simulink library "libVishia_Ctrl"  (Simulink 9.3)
settings: Solver=ode45  StartTime=0.0  StopTime=10.0  RelTol=1e-3  EnableMultiTasking=on
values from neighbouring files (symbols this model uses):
  Tstep = 0.0001    [InspcCtrl_init.m]    (also in TestOrthOscObjO_init.m = 0.0005; stimuli_Smlk.m = 0.001; TestOrthOsc_init.m = 5e-05; Test_PIDctrl_init.m)
undefined symbols (not defined in the file or in its folder): Fmax, Fmin, Fnom, init, K, lim, maxError, minMagn, T1, Td, Tg, TP, Tstep_, y0
libraries: $bdroot x14, libVishia_Conv x8, simulink x5, lib_Inspc x1

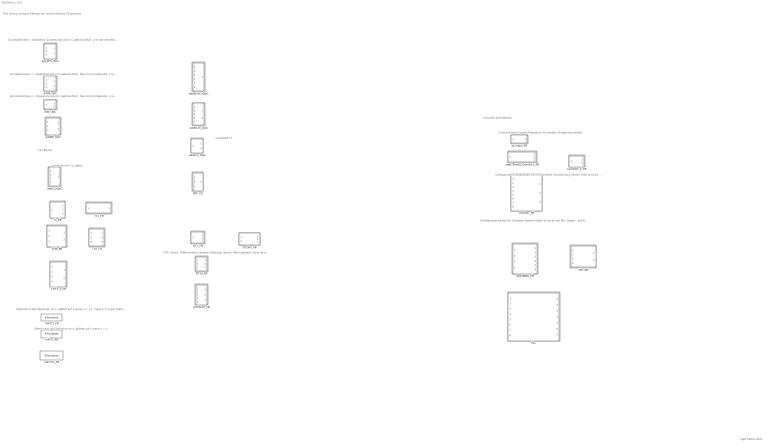
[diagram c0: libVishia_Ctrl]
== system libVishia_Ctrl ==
  note: right botton 60%
  note: Converts from a given Frequency to number of steps per period
  note: Simulink-pure Moduls
  note: This library contains FBlocks for control without S-Functions
  note: Orthogonaloszillator für 3-phasen-System Input ist als ab mit Mit- Gegen- und Nullsystem gegeben. Orthi separiert Gleichanteil (yG), Mitsystem(yM) und Gegensystem (yN) date=2016-03-04
  note: OrthogonalOscillator Basic-FB mit korrekter Rückführung. Dieser Orthi wird als Basis in den anderen FB verwendet.
  note: Grundglied des += Operators wie in C gebräuchlich. Das ist ein Integrator. y ist der neueste Wert. yz ist der gespeicherte Wert (Abarbeitung bevor +=). Ohne Setz-Möglichkeit. Initialwert als Parameter.
  note: Grundglied des += Operators wie in C gebräuchlich. Das ist ein Integrator. y ist der neueste Wert. yz ist der gespeicherte Wert (Abarbeitung bevor +=). Setzen: Wird in C häufig an anderer Stelle ausgeführt.
  note: Grundglied des = Operators (Zuweisung) wie in C gebräuchlich. y ist der neueste Wert, entweder =X oder =XS. yz ist der gespeicherte Wert. Setzen: Wird in C häufig an anderer Stelle ausgeführt.
  note: Variante mit z-1 außen.
  note: T1-FBlocks
  note: Übernimmt das Maximum an x, glättet auf x wenn x < y 1. Input x, 2. Input Faktor zum Glätten
  note: Übernimmt das Minimum an x, glättet auf x wenn x > y
  note: Limitated T1
  note: DT1 classic: Differenzierer, danach Glättung. Vorteil: Wenn gesetzt, dann ist das Differnzial 0
  DFF_CE : Subsystem
  DT1SLim_FB : Subsystem
  DT1S_FB : Subsystem
  DT1_FB : Subsystem
  DT1lim_FB : Subsystem
  OrthOsc_FB : Subsystem
  OrthiMNG_FB : Subsystem
  PLL : Subsystem
  T11_FB : Subsystem
  T1D_FB : Subsystem
  T1_FB : Subsystem
  T1fS_FB : Subsystem
  T1fT1_S_FB : Subsystem
  abn2pq : Subsystem
  addLim_OpC : Subsystem
  addSE_OpC : Subsystem  TreatAsAtomicUnit=on
  addSLim_OpC : Subsystem
  addSLim_zOpC : Subsystem
  addS_OpC : Subsystem
  addS_zOpC : Subsystem
  add_OpC : Subsystem
  assignS_OpC : Subsystem
  calcOrthi_fi_FB : Subsystem
  fq_steps_FB : Subsystem
  maxT1_FB : S-Function  FunctionName=maxT1_FB  Parameters=SampleTime  SFunctionDeploymentMode=off  EnableBusSupport=off
  maxnT1_FB : S-Function  FunctionName=maxnT1_FB  Parameters=SampleTime  SFunctionDeploymentMode=off  EnableBusSupport=off
  minT1_FB : S-Function  FunctionName=minT1_FB  Parameters=SampleTime  SFunctionDeploymentMode=off  EnableBusSupport=off
  step7Period_OrthOsc1_FB : Subsystem

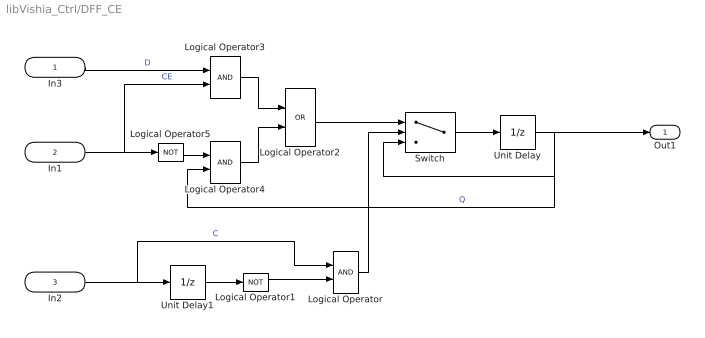
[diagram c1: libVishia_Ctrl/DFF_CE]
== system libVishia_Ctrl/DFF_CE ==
  In3 : Inport
  In1 : Inport  Port=2
  In2 : Inport  Port=3
  Logical Operator : Logic  IconShape=distinctive  AllPortsSameDT=off  OutDataTypeStr=boolean
  Logical Operator1 : Logic  Operator=NOT  IconShape=distinctive  AllPortsSameDT=off  OutDataTypeStr=boolean
  Logical Operator2 : Logic  Operator=OR  IconShape=distinctive  AllPortsSameDT=off  OutDataTypeStr=boolean
  Logical Operator3 : Logic  IconShape=distinctive  AllPortsSameDT=off  OutDataTypeStr=boolean
  Logical Operator4 : Logic  IconShape=distinctive  AllPortsSameDT=off  OutDataTypeStr=boolean
  Logical Operator5 : Logic  Operator=NOT  IconShape=distinctive  AllPortsSameDT=off  OutDataTypeStr=boolean
  Switch : Switch  Criteria=u2 > Threshold
  Unit Delay : UnitDelay  SampleTime=-1  HasFrameUpgradeWarning=on
  Unit Delay1 : UnitDelay  SampleTime=-1  HasFrameUpgradeWarning=on
  Out1 : Outport  OutDataTypeStr=boolean
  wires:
  In1/1 -> Logical Operator3/2, Logical Operator5/1  "CE"
  Switch/1 -> Unit Delay/1
  In2/1 -> Logical Operator/1, Unit Delay1/1  "C"
  Unit Delay1/1 -> Logical Operator1/1
  Logical Operator1/1 -> Logical Operator/2
  Logical Operator/1 -> Switch/2
  Unit Delay/1 -> Logical Operator4/2, Switch/3, Out1/1  "Q"
  In3/1 -> Logical Operator3/1  "D"
  Logical Operator5/1 -> Logical Operator4/1
  Logical Operator2/1 -> Switch/1
  Logical Operator4/1 -> Logical Operator2/2
  Logical Operator3/1 -> Logical Operator2/1

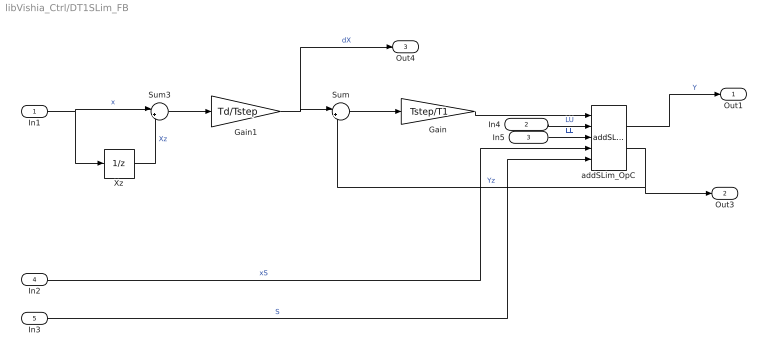
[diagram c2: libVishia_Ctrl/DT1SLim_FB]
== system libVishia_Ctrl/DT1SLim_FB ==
  In1 : Inport
  In4 : Inport  Port=2
  In5 : Inport  Port=3
  In2 : Inport  Port=4
  In3 : Inport  Port=5
  Gain : Gain  Gain=Tstep/T1
  Gain1 : Gain  Gain=Td/Tstep
  Sum : Sum  Inputs=|+-
  Sum3 : Sum  Inputs=|+-
  Xz : UnitDelay  SampleTime=Tstep  HasFrameUpgradeWarning=on
  addSLim_OpC : $bdroot/addSLim_OpC  y0=0  Tstep=Tstep
  Out1 : Outport
  Out3 : Outport  Port=2
  Out4 : Outport  Port=3
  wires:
  addSLim_OpC/2 -> Out3/1, Sum/2  "Yz"
  In3/1 -> addSLim_OpC/5  "S"
  In2/1 -> addSLim_OpC/4  "xS"
  Sum3/1 -> Gain1/1
  Xz/1 -> Sum3/2  "Xz"
  Gain1/1 -> Sum/1, Out4/1  "dX"
  addSLim_OpC/1 -> Out1/1  "Y"
  In1/1 -> Sum3/1, Xz/1  "x"
  Sum/1 -> Gain/1
  Gain/1 -> addSLim_OpC/1
  In4/1 -> addSLim_OpC/2  "LU"
  In5/1 -> addSLim_OpC/3  "LL"

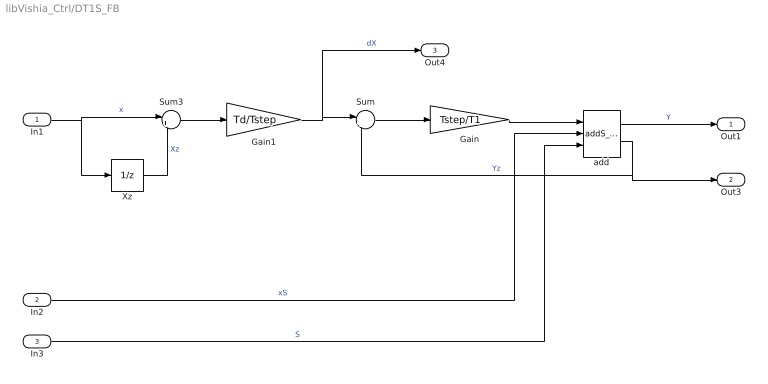
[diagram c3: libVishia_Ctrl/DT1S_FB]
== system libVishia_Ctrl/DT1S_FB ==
  In1 : Inport
  In2 : Inport  Port=2
  In3 : Inport  Port=3
  Gain : Gain  Gain=Tstep/T1
  Gain1 : Gain  Gain=Td/Tstep
  Sum : Sum  Inputs=|+-
  Sum3 : Sum  Inputs=|+-
  Xz : UnitDelay  SampleTime=Tstep  HasFrameUpgradeWarning=on
  add : $bdroot/addS_OpC  init=0  Tstep=Tstep
  Out1 : Outport
  Out3 : Outport  Port=2
  Out4 : Outport  Port=3
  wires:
  Gain/1 -> add/1
  Sum/1 -> Gain/1
  In1/1 -> Xz/1, Sum3/1  "x"
  add/1 -> Out1/1  "Y"
  Gain1/1 -> Out4/1, Sum/1  "dX"
  Xz/1 -> Sum3/2  "Xz"
  Sum3/1 -> Gain1/1
  In2/1 -> add/2  "xS"
  In3/1 -> add/3  "S"
  add/2 -> Sum/2, Out3/1  "Yz"

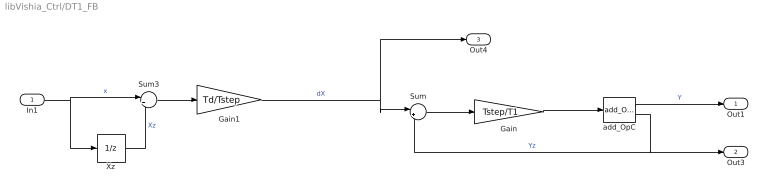
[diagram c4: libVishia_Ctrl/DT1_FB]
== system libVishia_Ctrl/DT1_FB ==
  In1 : Inport
  Gain : Gain  Gain=Tstep/T1
  Gain1 : Gain  Gain=Td/Tstep
  Sum : Sum  Inputs=|+-
  Sum3 : Sum  Inputs=|+-
  Xz : UnitDelay  SampleTime=Tstep  HasFrameUpgradeWarning=on
  add_OpC : $bdroot/add_OpC  y0=0  Tstep=Tstep
  Out1 : Outport
  Out3 : Outport  Port=2
  Out4 : Outport  Port=3
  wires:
  add_OpC/2 -> Out3/1, Sum/2  "Yz"
  Sum3/1 -> Gain1/1
  Xz/1 -> Sum3/2  "Xz"
  add_OpC/1 -> Out1/1  "Y"
  In1/1 -> Sum3/1, Xz/1  "x"
  Sum/1 -> Gain/1
  Gain/1 -> add_OpC/1
  Gain1/1 -> Sum/1, Out4/1  "dX"

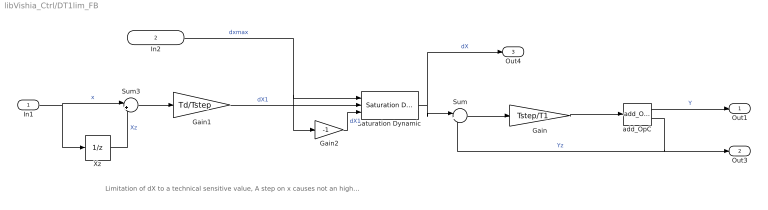
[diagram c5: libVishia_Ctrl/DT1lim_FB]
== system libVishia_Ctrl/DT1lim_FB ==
  note: Limitation of dX to a technical sensitive value, A step on x causes not an higher value on dX1, which is smoothed. So fast changes are filtered.
  In1 : Inport
  In2 : Inport  Port=2
  Gain : Gain  Gain=Tstep/T1
  Gain1 : Gain  Gain=Td/Tstep
  Gain2 : Gain  Gain=-1
  Saturation Dynamic : simulink/Discontinuities/Saturation Dynamic  OutMin=[]  OutMax=[]  OutDataTypeStr=Inherit: Same as second input  OutDataType=fixdt(1, 16)  OutScaling=2^-10  DoSatur=off
  Sum : Sum  Inputs=|+-
  Sum3 : Sum  Inputs=|+-
  Xz : UnitDelay  SampleTime=Tstep  HasFrameUpgradeWarning=on
  add_OpC : $bdroot/add_OpC  y0=0  Tstep=Tstep
  Out1 : Outport
  Out3 : Outport  Port=2
  Out4 : Outport  Port=3
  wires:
  Saturation Dynamic/1 -> Out4/1, Sum/1  "dX"
  Gain/1 -> add_OpC/1
  Sum/1 -> Gain/1
  In1/1 -> Xz/1, Sum3/1  "x"
  add_OpC/1 -> Out1/1  "Y"
  Gain1/1 -> Saturation Dynamic/2  "dX1"
  Xz/1 -> Sum3/2  "Xz"
  Sum3/1 -> Gain1/1
  add_OpC/2 -> Sum/2, Out3/1  "Yz"
  In2/1 -> Gain2/1, Saturation Dynamic/1  "dxmax"
  Gain2/1 -> Saturation Dynamic/3  "dX1"

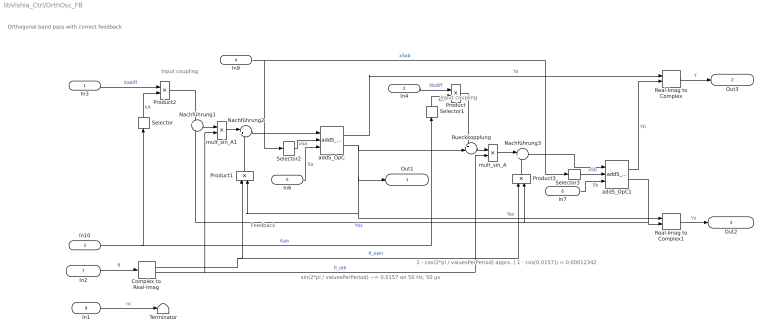
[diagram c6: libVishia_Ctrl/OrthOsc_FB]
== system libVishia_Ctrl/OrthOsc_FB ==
  note: 1 - cos(2*pi / valuesPerPeriod) apprx. ( 1 - cos(0.0157)) = 0.00012342
  note: Input coupling
  note: Feedback
  note: sin(2*pi / valuesPerPeriod) ~= 0.0157 on 50 Hz, 50 µs
  note: Orthogonal band pass with correct feedback
  note: Input coupling
  In3 : Inport
  In4 : Inport  Port=2
  In10 : Inport  Port=3  OutDataTypeStr=single  PortDimensions=2
  In9 : Inport  Port=4
  In6 : Inport  Port=5  OutDataTypeStr=boolean
  In7 : Inport  Port=6  OutDataTypeStr=boolean
  In2 : Inport  Port=7  OutDataTypeStr=single
  In1 : Inport  Port=8  OutDataTypeStr=boolean
  Complex to Real-Imag : ComplexToRealImag
  Nachführung1 : Sum  Inputs=+|-
  Nachführung2 : Sum  Inputs=|+-
  Nachführung3 : Sum  Inputs=|+-
  Product{,1..3} (4 alike) : Product
  Real-Imag to Complex : RealImagToComplex
  Real-Imag to Complex1 : RealImagToComplex
  Rueckkopplung : Sum  Inputs=++|
  Selector : Selector  InputPortWidth=2  IndexOptions=Index vector (dialog)  Indices=[1]  OutputSizes=1
  Selector1 : Selector  InputPortWidth=2  IndexOptions=Index vector (dialog)  Indices=[2]  OutputSizes=1
  Selector2 : Selector  InputPortWidth=2  IndexOptions=Index vector (dialog)  Indices=[1]  OutputSizes=1
  Selector3 : Selector  InputPortWidth=2  IndexOptions=Index vector (dialog)  Indices=[2]  OutputSizes=1
  Terminator : Terminator
  addS_OpC : $bdroot/addS_OpC  init=0  Tstep=-1
  addS_OpC1 : $bdroot/addS_OpC  init=0  Tstep=-1
  mult_sin_A : Product
  mult_sin_A1 : Product
  Out1 : Outport
  Out3 : Outport  Port=2
  Out2 : Outport  Port=3
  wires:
  Complex to Real-Imag/2 -> mult_sin_A1/2, mult_sin_A/2  "fI_oth"
  Real-Imag to Complex/1 -> Out3/1  "Y"
  mult_sin_A1/1 -> Nachführung2/1
  Nachführung1/1 -> mult_sin_A1/1
  addS_OpC/2 -> Out1/1, Real-Imag to Complex1/1, Product1/2, Rueckkopplung/2  "Yaz"
  Product2/1 -> Nachführung1/1
  In3/1 -> Product2/1  "Xadiff"
  Product/1 -> Rueckkopplung/1
  In2/1 -> Complex to Real-Imag/1  "fI"
  Rueckkopplung/1 -> mult_sin_A/1
  mult_sin_A/1 -> Nachführung3/1
  addS_OpC/1 -> Real-Imag to Complex/1  "Ya"
  addS_OpC1/2 -> Nachführung1/2, Product3/2, Real-Imag to Complex1/2  "Ybz"
  Selector/1 -> Product2/2  "kA"
  In6/1 -> addS_OpC/3  "Sa"
  In4/1 -> Product/1  "Xbdiff"
  Selector1/1 -> Product/2  "kB"
  In7/1 -> addS_OpC1/3  "Sb"
  Selector3/1 -> addS_OpC1/2  "xSb"
  Selector2/1 -> addS_OpC/2  "xSA"
  Nachführung2/1 -> addS_OpC/1
  Product1/1 -> Nachführung2/2
  Nachführung3/1 -> addS_OpC1/1
  Product3/1 -> Nachführung3/2
  Complex to Real-Imag/1 -> Product1/1, Product3/1  "fI_own"
  addS_OpC1/1 -> Real-Imag to Complex/2  "Yb"
  Real-Imag to Complex1/1 -> Out2/1  "Yz"
  In10/1 -> Selector/1, Selector1/1  "Kab"
  In9/1 -> Selector3/1, Selector2/1  "xSab"
  In1/1 -> Terminator/1  "nc"

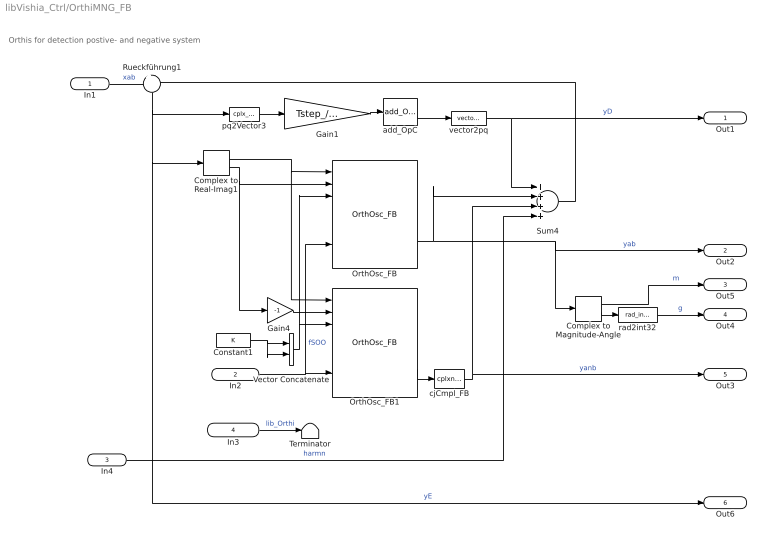
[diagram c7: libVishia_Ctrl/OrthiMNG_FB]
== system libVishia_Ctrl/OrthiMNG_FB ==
  note: Orthis for detection postive- and negative system
  In1 : Inport  OutDataTypeStr=single
  In2 : Inport  Port=2  OutDataTypeStr=single
  In4 : Inport  Port=3  OutDataTypeStr=single
  In3 : Inport  Port=4  OutDataTypeStr=boolean
  Complex to Magnitude-Angle : ComplexToMagnitudeAngle
  Complex to Real-Imag1 : ComplexToRealImag
  Constant1 : Constant  Value=K  OutDataTypeStr=single
  Gain1 : Gain  Gain=Tstep_/Tg
  Gain4 : Gain  Gain=-1
  OrthOsc_FB : $bdroot/OrthOsc_FB
  OrthOsc_FB1 : $bdroot/OrthOsc_FB
  Rueckführung1 : Sum  Inputs=+-
  Sum4 : Sum  Inputs=++++
  Terminator : Terminator
  Vector Concatenate : Concatenate
  add_OpC : $bdroot/add_OpC  y0=0  Tstep=-1
  cjCmpl_FB : libVishia_Conv/cplxni_FB  SystemSampleTime=-1
  pq2Vector3 : libVishia_Conv/cplx_vector_FB  SystemSampleTime=-1
  rad2int32 : libVishia_Conv/rad_int32_FB  SystemSampleTime=-1
  vector2pq : libVishia_Conv/vector_cplx_FB  SystemSampleTime=-1
  Out1 : Outport  OutDataTypeStr=single
  Out2 : Outport  Port=2  OutDataTypeStr=single
  Out5 : Outport  Port=3  OutDataTypeStr=single
  Out4 : Outport  Port=4  OutDataTypeStr=int32
  Out3 : Outport  Port=5  OutDataTypeStr=single
  Out6 : Outport  Port=6  OutDataTypeStr=single
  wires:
  In4/1 -> Sum4/4  "harmn"
  In3/1 -> Terminator/1  "lib_Orthi"
  Constant1/1 -> Vector Concatenate/1, Vector Concatenate/2
  Gain4/1 -> OrthOsc_FB1/2
  Complex to Real-Imag1/2 -> OrthOsc_FB/2, Gain4/1
  add_OpC/2 -> vector2pq/1
  pq2Vector3/1 -> Gain1/1
  Complex to Real-Imag1/1 -> OrthOsc_FB/1, OrthOsc_FB1/1
  vector2pq/1 -> Out1/1, Sum4/1  "yD"
  Vector Concatenate/1 -> OrthOsc_FB/3, OrthOsc_FB1/3
  Rueckführung1/1 -> pq2Vector3/1, Complex to Real-Imag1/1, Out6/1  "yE"
  In1/1 -> Rueckführung1/1  "xab"
  Gain1/1 -> add_OpC/1
  In2/1 -> OrthOsc_FB1/7, OrthOsc_FB/7  "fSOO"
  OrthOsc_FB/3 -> Complex to Magnitude-Angle/1, Out2/1, Sum4/2  "yab"
  Sum4/1 -> Rueckführung1/2
  cjCmpl_FB/1 -> Out3/1, Sum4/3  "yanb"
  OrthOsc_FB1/3 -> cjCmpl_FB/1
  Complex to Magnitude-Angle/2 -> rad2int32/1
  rad2int32/1 -> Out4/1  "g"
  Complex to Magnitude-Angle/1 -> Out5/1  "m"

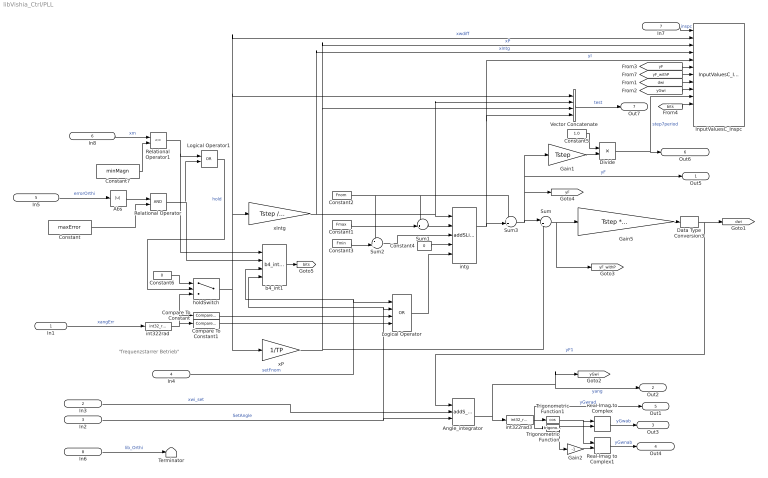
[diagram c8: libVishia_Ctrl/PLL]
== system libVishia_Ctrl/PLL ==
  note: "frequenzstarrer Betrieb"
  In1 : Inport
  In3 : Inport  Port=2  OutDataTypeStr=int32
  In2 : Inport  Port=3  OutDataTypeStr=boolean
  In4 : Inport  Port=4  OutDataTypeStr=boolean
  In5 : Inport  Port=5  OutDataTypeStr=single  PortDimensions=1
  In8 : Inport  Port=6  OutDataTypeStr=single  PortDimensions=1
  In7 : Inport  Port=7  OutDataTypeStr=uint32  PortDimensions=1  SampleTime=Tstep
  In6 : Inport  Port=8  OutDataTypeStr=boolean
  Abs : Abs
  Angle_integrator : $bdroot/addS_OpC  init=0  Tstep=-1
  Compare To Constant : simulink/Logic and Bit Operations/Compare To Constant  relop=>=  const=0.1  OutDataTypeStr=boolean
  Compare To Constant1 : simulink/Logic and Bit Operations/Compare To Constant  relop=<  const=-0.1  OutDataTypeStr=boolean
  Constant : Constant  Value=maxError
  Constant1 : Constant  Value=Fmax  OutDataTypeStr=single
  Constant2 : Constant  Value=Fnom  OutDataTypeStr=single
  Constant3 : Constant  Value=Fmin  OutDataTypeStr=single
  Constant4 : Constant  Value=0  OutDataTypeStr=single
  Constant5 : Constant  Value=1.0  OutDataTypeStr=single
  Constant6 : Constant  Value=0  OutDataTypeStr=single
  Constant7 : Constant  Value=minMagn
  Data Type Conversion3 : DataTypeConversion  OutDataTypeStr=int32
  Divide : Product  Inputs=*/
  Gain1 : Gain  Gain=Tstep
  Gain2 : Gain  Gain=-1
  Gain5 : Gain  Gain=Tstep * 65536 * 65536
  InputValuesC_Inspc : lib_Inspc/InputValuesC_Inspc  Commented=on  nameRefl=nameInspc  n1='wxdiff_rad'  n2='xP'  n3='xIntg'  n4='yIntg'  n5='yF'  n6='yF_withP'  n7='dwi'  n8='yGwi'  n9='step7period'  n10='hold_setG_setF_err_magn'  n11=''  n12=''
  Logical Operator : Logic  Operator=OR  Inputs=4  IconShape=distinctive  AllPortsSameDT=off  OutDataTypeStr=boolean
  Logical Operator1 : Logic  Operator=OR  AllPortsSameDT=off  OutDataTypeStr=boolean
  Real-Imag to Complex : RealImagToComplex
  Real-Imag to Complex1 : RealImagToComplex
  Relational Operator : RelationalOperator  OutDataTypeStr=boolean
  Relational Operator1 : RelationalOperator  Operator=<=  OutDataTypeStr=boolean
  Sum : Sum  Inputs=|++
  Sum1 : Sum  Inputs=-+|
  Sum2 : Sum  Inputs=-+|
  Sum3 : Sum  Inputs=++|
  Terminator : Terminator
  Trigonometric Function : Trigonometry
  Trigonometric Function1 : Trigonometry  Operator=cos
  Vector Concatenate : Concatenate  NumInputs=4
  b4_int1 : libVishia_Conv/b4_int32_FB  b0bit=0  b1bit=1  b2bit=2  b3bit=3
  holdSwitch : Switch
  int322rad : libVishia_Conv/int32_rad_FB  SystemSampleTime=-1
  int322rad3 : libVishia_Conv/int32_rad_FB  SystemSampleTime=-1
  intg : $bdroot/addSLim_OpC  y0=0  Tstep=-1
  xIntg : Gain  Gain=Tstep / Tintg
  xP : Gain  Gain=1/TP
  Out5 : Outport  OutDataTypeStr=single  PortDimensions=1
  Out2 : Outport  Port=2  OutDataTypeStr=int32  PortDimensions=1
  Out3 : Outport  Port=3  OutDataTypeStr=single  PortDimensions=1
  Out4 : Outport  Port=4  OutDataTypeStr=single  PortDimensions=1
  Out1 : Outport  Port=5  OutDataTypeStr=single  PortDimensions=1
  Out6 : Outport  Port=6  OutDataTypeStr=single  PortDimensions=1
  Out7 : Outport  Port=7  OutDataTypeStr=single  PortDimensions=4
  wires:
  [bits] -> InputValuesC_Inspc/11
  b4_int1/1 -> [bits]
  [yF] -> InputValuesC_Inspc/6
  In8/1 -> Relational Operator1/1  "xm"
  Relational Operator/1 -> b4_int1/2, Logical Operator1/2
  Relational Operator1/1 -> b4_int1/1, Logical Operator1/1
  Constant7/1 -> Relational Operator1/2
  Constant/1 -> Relational Operator/2
  Abs/1 -> Relational Operator/1
  In5/1 -> Abs/1  "errorOrthi"
  [yGwi] -> InputValuesC_Inspc/9
  [dwi] -> InputValuesC_Inspc/8
  [yF_withP] -> InputValuesC_Inspc/7
  In7/1 -> InputValuesC_Inspc/1  "inspc"
  int322rad/1 -> Compare To Constant1/1, holdSwitch/3, Compare To Constant/1
  Constant6/1 -> holdSwitch/1
  Vector Concatenate/1 -> Out7/1  "test"
  In6/1 -> Terminator/1  "lib_Orthi"
  holdSwitch/1 -> Vector Concatenate/1, InputValuesC_Inspc/2, xIntg/1, xP/1  "xwdiff"
  Logical Operator1/1 -> holdSwitch/2  "hold"
  In4/1 -> Logical Operator/1, b4_int1/3  "setFnom"
  Logical Operator/1 -> intg/5
  Divide/1 -> Out6/1, InputValuesC_Inspc/10  "step7period"
  Constant5/1 -> Divide/1
  Gain1/1 -> Divide/2
  In3/1 -> Angle_integrator/2  "xwi_set"
  In2/1 -> b4_int1/4, Logical Operator/2, Angle_integrator/3  "SetAngle"
  xIntg/1 -> Vector Concatenate/2, intg/1, InputValuesC_Inspc/4  "xIntg"
  xP/1 -> Sum/2, Vector Concatenate/3, InputValuesC_Inspc/3  "xP"
  In1/1 -> int322rad/1  "xangErr"
  Constant4/1 -> intg/4
  Constant3/1 -> Sum2/2
  Sum2/1 -> intg/3
  Sum1/1 -> intg/2
  Constant2/1 -> Sum3/1, Sum1/1, Sum2/1
  Sum/1 -> Gain5/1, [yF_withP]
  Data Type Conversion3/1 -> Angle_integrator/1, [dwi]  "yF1"
  Constant1/1 -> Sum1/2
  intg/1 -> Sum3/2, Vector Concatenate/4, InputValuesC_Inspc/5  "yI"
  Gain5/1 -> Data Type Conversion3/1
  Real-Imag to Complex1/1 -> Out4/1  "yGwnab"
  Real-Imag to Complex/1 -> Out3/1  "yGwab"
  Gain2/1 -> Real-Imag to Complex1/2
  Trigonometric Function/1 -> Real-Imag to Complex/2, Gain2/1
  Trigonometric Function1/1 -> Real-Imag to Complex/1, Real-Imag to Complex1/1
  int322rad3/1 -> Trigonometric Function1/1, Trigonometric Function/1, Out1/1  "yGwrad"
  Angle_integrator/2 -> int322rad3/1, Out2/1, [yGwi]  "yang"
  Sum3/1 -> Out5/1, Gain1/1, [yF], Sum/1  "yF"
  Compare To Constant/1 -> Logical Operator/3
  Compare To Constant1/1 -> Logical Operator/4

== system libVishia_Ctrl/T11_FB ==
  note: Yz += Tstep/T1 * (x - Yz)
  In1 : Inport
  Gain : Gain  Gain=Tstep/T1
  Sum : Sum  Inputs=|+-
  Sum6 : Sum  Inputs=|++
  Unit Delay : UnitDelay  InitialCondition=y0  SampleTime=Tstep  HasFrameUpgradeWarning=on
  Out2 : Outport
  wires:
  In1/1 -> Sum/1  "X"
  Sum/1 -> Gain/1  "dT1_Y"
  Gain/1 -> Sum6/1
  Sum6/1 -> Unit Delay/1
  Unit Delay/1 -> Sum/2, Sum6/2, Out2/1  "y"

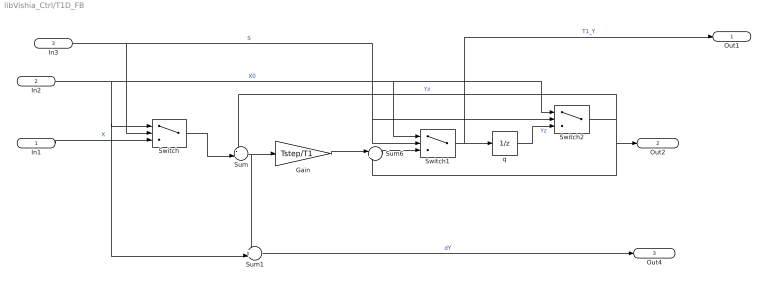
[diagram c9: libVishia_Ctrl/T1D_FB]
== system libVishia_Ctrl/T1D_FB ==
  In1 : Inport
  In2 : Inport  Port=2
  In3 : Inport  Port=3
  Gain : Gain  Gain=Tstep/T1
  Sum : Sum  Inputs=-+|
  Sum1 : Sum  Inputs=++|
  Sum6 : Sum  Inputs=|++
  Switch : Switch  Criteria=u2 ~= 0
  Switch1 : Switch  Criteria=u2 ~= 0
  Switch2 : Switch  Criteria=u2 ~= 0
  q : UnitDelay  InitialCondition=y0  SampleTime=Tstep  HasFrameUpgradeWarning=on
  Out1 : Outport
  Out2 : Outport  Port=2
  Out4 : Outport  Port=3
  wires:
  Switch2/1 -> Sum6/2, Out2/1, Sum/1  "Yz"
  Switch1/1 -> Out1/1, q/1  "T1_Y"
  In1/1 -> Switch/3  "X"
  In2/1 -> Sum1/2, Switch/1, Switch1/1, Switch2/1  "X0"
  Sum/1 -> Gain/1, Sum1/1
  In3/1 -> Switch/2, Switch2/2, Switch1/2  "S"
  Switch/1 -> Sum/2
  Sum1/1 -> Out4/1  "dY"
  Gain/1 -> Sum6/1
  Sum6/1 -> Switch1/3
  q/1 -> Switch2/3  "Yz"

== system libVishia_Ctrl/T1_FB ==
  note: Yz += Tstep/T1 * (x - Yz)
  In1 : Inport
  Gain : Gain  Gain=Tstep/T1
  Sum : Sum  Inputs=|+-
  add_OpC : $bdroot/add_OpC  y0=y0  Tstep=-1
  Out1 : Outport
  Out2 : Outport  Port=2
  Out4 : Outport  Port=3
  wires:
  Gain/1 -> add_OpC/1
  Sum/1 -> Out4/1, Gain/1  "dT1_Y"
  In1/1 -> Sum/1  "X"
  add_OpC/1 -> Out1/1  "T1_Y"
  add_OpC/2 -> Out2/1, Sum/2  "Yz"

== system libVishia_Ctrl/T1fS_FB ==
  In1 : Inport
  In2 : Inport  Port=2
  In3 : Inport  Port=3  OutDataTypeStr=boolean
  Gain : Gain  Gain=Tstep/T1
  Sum : Sum  Inputs=|+-
  addS_OpC : $bdroot/addS_OpC  init=init  Tstep=Tstep
  Out1 : Outport
  Out2 : Outport  Port=2
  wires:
  Gain/1 -> addS_OpC/1
  Sum/1 -> Gain/1
  In1/1 -> Sum/1  "x"
  addS_OpC/1 -> Out1/1  "Y"
  addS_OpC/2 -> Out2/1, Sum/2  "Yz"
  In2/1 -> addS_OpC/2  "xS"
  In3/1 -> addS_OpC/3  "S"

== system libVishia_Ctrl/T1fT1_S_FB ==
  In1 : Inport
  In4 : Inport  Port=2
  In2 : Inport  Port=3
  In3 : Inport  Port=4  OutDataTypeStr=boolean
  Gain : Gain  Gain=Tstep/T1
  Product : Product
  Sum : Sum  Inputs=|+-
  addS_OpC : $bdroot/addS_OpC  init=y0  Tstep=Tstep
  Out1 : Outport
  Out2 : Outport  Port=2
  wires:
  In3/1 -> addS_OpC/3  "S"
  In2/1 -> addS_OpC/2  "xS"
  addS_OpC/2 -> Sum/2, Out2/1  "Yz"
  addS_OpC/1 -> Out1/1  "Y_T1"
  In1/1 -> Sum/1  "x"
  Sum/1 -> Gain/1
  Product/1 -> addS_OpC/1
  In4/1 -> Product/1  "fT1"
  Gain/1 -> Product/2

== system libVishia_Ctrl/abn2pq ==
  note: Park transformation of positive and negativ system
  In1 : Inport  OutDataTypeStr=single
  In2 : Inport  Port=2  OutDataTypeStr=single
  In4 : Inport  Port=3  OutDataTypeStr=single
  In3 : Inport  Port=4  OutDataTypeStr=boolean
  Product : Product
  Product1 : Product
  Terminator : Terminator
  cplxni_FB : libVishia_Conv/cplxni_FB  SystemSampleTime=-1
  Out4 : Outport  OutDataTypeStr=single
  Out5 : Outport  Port=2  OutDataTypeStr=single
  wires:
  In3/1 -> Terminator/1  "lib_OrthOsc"
  In1/1 -> Product/1  "ab"
  In2/1 -> Product1/1  "abN"
  cplxni_FB/1 -> Product/2
  In4/1 -> cplxni_FB/1, Product1/2  "xgab"
  Product/1 -> Out4/1  "ypq"
  Product1/1 -> Out5/1  "ypqN"

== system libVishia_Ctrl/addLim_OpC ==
  x : Inport
  Saturation : Saturate  UpperLimit=lim  LowerLimit=-lim
  Sum6 : Sum  Inputs=|++
  Unit Delay : UnitDelay  InitialCondition=y0  SampleTime=Tstep  HasFrameUpgradeWarning=on
  y : Outport
  yz : Outport  Port=2
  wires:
  Unit Delay/1 -> Sum6/2, yz/1
  x/1 -> Sum6/1
  Saturation/1 -> y/1, Unit Delay/1
  Sum6/1 -> Saturation/1

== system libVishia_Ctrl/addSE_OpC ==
  x : Inport
  xS : Inport  Port=2
  S : Inport  Port=3  OutDataTypeStr=boolean
  Enable : EnablePort
  Sum6 : Sum  Inputs=|++
  Switch : Switch  Criteria=u2 ~= 0
  q : UnitDelay  SampleTime=-1  HasFrameUpgradeWarning=on
  y : Outport
  yz : Outport  Port=2
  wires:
  Switch/1 -> q/1, y/1
  x/1 -> Sum6/1
  q/1 -> Sum6/2, yz/1
  S/1 -> Switch/2
  Sum6/1 -> Switch/3
  xS/1 -> Switch/1

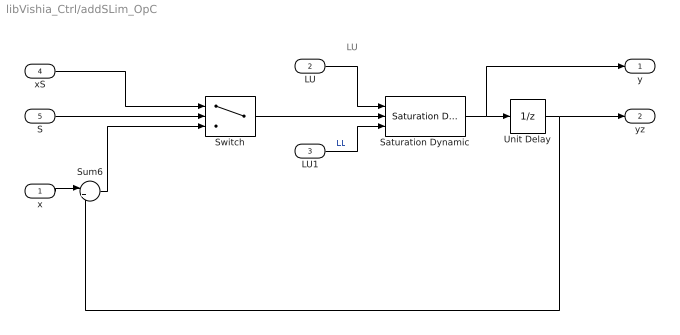
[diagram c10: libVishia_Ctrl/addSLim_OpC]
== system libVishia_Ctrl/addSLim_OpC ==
  note: LU
  x : Inport
  LU : Inport  Port=2
  LU1 : Inport  Port=3
  xS : Inport  Port=4
  S : Inport  Port=5  OutDataTypeStr=boolean
  Saturation Dynamic : simulink/Discontinuities/Saturation Dynamic  OutMin=[]  OutMax=[]  OutDataTypeStr=Inherit: Same as second input  OutDataType=fixdt(1, 16)  OutScaling=2^-10  DoSatur=off
  Sum6 : Sum  Inputs=|++
  Switch : Switch  Criteria=u2 ~= 0
  Unit Delay : UnitDelay  InitialCondition=y0  SampleTime=Tstep  HasFrameUpgradeWarning=on
  y : Outport
  yz : Outport  Port=2
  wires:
  Switch/1 -> Saturation Dynamic/2
  S/1 -> Switch/2
  Unit Delay/1 -> yz/1, Sum6/2
  xS/1 -> Switch/1
  x/1 -> Sum6/1
  Sum6/1 -> Switch/3
  Saturation Dynamic/1 -> y/1, Unit Delay/1
  LU/1 -> Saturation Dynamic/1
  LU1/1 -> Saturation Dynamic/3  "LL"

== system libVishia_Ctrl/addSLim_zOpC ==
  note: LU
  x : Inport
  LU : Inport  Port=2
  LU1 : Inport  Port=3
  xS : Inport  Port=4
  S : Inport  Port=5  OutDataTypeStr=boolean
  yz : Inport  Port=6
  Saturation Dynamic : simulink/Discontinuities/Saturation Dynamic  OutMin=[]  OutMax=[]  OutDataTypeStr=Inherit: Same as second input  OutDataType=fixdt(1, 16)  OutScaling=2^-10  DoSatur=off
  Sum6 : Sum  Inputs=|++
  Switch : Switch  Criteria=u2 ~= 0
  y : Outport
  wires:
  LU1/1 -> Saturation Dynamic/3  "LL"
  LU/1 -> Saturation Dynamic/1
  Saturation Dynamic/1 -> y/1  "y"
  Sum6/1 -> Switch/3
  x/1 -> Sum6/1
  xS/1 -> Switch/1
  S/1 -> Switch/2
  Switch/1 -> Saturation Dynamic/2
  yz/1 -> Sum6/2  "yz"

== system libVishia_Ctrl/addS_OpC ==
  x : Inport
  xS : Inport  Port=2
  S : Inport  Port=3  OutDataTypeStr=boolean
  Sum6 : Sum  Inputs=|++
  Switch : Switch  Criteria=u2 ~= 0
  q : UnitDelay  InitialCondition=init  SampleTime=Tstep  HasFrameUpgradeWarning=on
  y : Outport
  yz : Outport  Port=2
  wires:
  Sum6/1 -> Switch/3
  x/1 -> Sum6/1
  xS/1 -> Switch/1
  q/1 -> Sum6/2, yz/1
  S/1 -> Switch/2
  Switch/1 -> q/1, y/1

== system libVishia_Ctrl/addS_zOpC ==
  x : Inport
  xS : Inport  Port=2
  S : Inport  Port=3  OutDataTypeStr=boolean
  yz : Inport  Port=4
  Sum6 : Sum  Inputs=|++
  Switch : Switch  Criteria=u2 ~= 0
  y : Outport
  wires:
  Switch/1 -> y/1
  S/1 -> Switch/2
  xS/1 -> Switch/1
  x/1 -> Sum6/1
  Sum6/1 -> Switch/3
  yz/1 -> Sum6/2  "yz"

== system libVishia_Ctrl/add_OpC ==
  x : Inport
  Delay : Delay  DelayLength=1  InitialCondition=y0  SampleTime=Tstep
  Sum6 : Sum  Inputs=|++
  y : Outport
  yz : Outport  Port=2
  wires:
  Sum6/1 -> Delay/1, y/1
  x/1 -> Sum6/1
  Delay/1 -> Sum6/2, yz/1

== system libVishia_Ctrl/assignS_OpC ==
  x : Inport
  xS : Inport  Port=2
  S : Inport  Port=3  OutDataTypeStr=boolean
  Switch : Switch  Criteria=u2 ~= 0
  Unit Delay : UnitDelay  InitialCondition=y0  SampleTime=Tstep  HasFrameUpgradeWarning=on
  y : Outport
  yz : Outport  Port=2
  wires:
  Switch/1 -> y/1, Unit Delay/1
  S/1 -> Switch/2
  Unit Delay/1 -> yz/1
  xS/1 -> Switch/1
  x/1 -> Switch/3

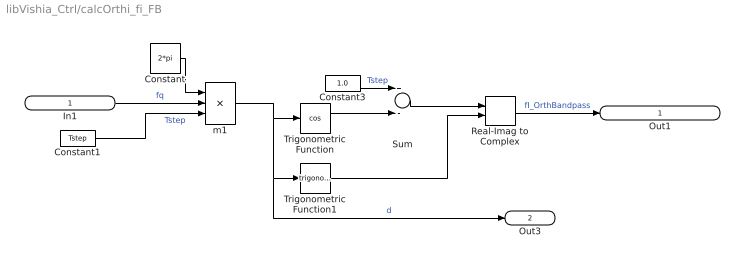
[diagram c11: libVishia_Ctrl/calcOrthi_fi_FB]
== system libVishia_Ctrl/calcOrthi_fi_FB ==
  In1 : Inport  OutDataTypeStr=single
  Constant : Constant  Value=2*pi  OutDataTypeStr=single
  Constant1 : Constant  Value=Tstep  OutDataTypeStr=single
  Constant3 : Constant  Value=1.0  OutDataTypeStr=single
  Real-Imag to Complex : RealImagToComplex
  Sum : Sum  Inputs=+-
  Trigonometric Function : Trigonometry  Operator=cos
  Trigonometric Function1 : Trigonometry
  m1 : Product  Inputs=***
  Out1 : Outport
  Out3 : Outport  Port=2
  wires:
  Sum/1 -> Real-Imag to Complex/1
  Trigonometric Function1/1 -> Real-Imag to Complex/2
  Real-Imag to Complex/1 -> Out1/1  "fI_OrthBandpass"
  In1/1 -> m1/2  "fq"
  m1/1 -> Out3/1, Trigonometric Function1/1, Trigonometric Function/1  "d"
  Constant/1 -> m1/1
  Constant1/1 -> m1/3  "Tstep"
  Trigonometric Function/1 -> Sum/2
  Constant3/1 -> Sum/1  "Tstep"

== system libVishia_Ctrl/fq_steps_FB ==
  fq : Inport
  Constant : Constant
  Data Type Duplicate : DataTypeDuplicate
  Data Type Conversion : DataTypeConversion
  Divide : Product  Inputs=*/
  Gain : Gain  Gain=Tstep
  nStep : Outport
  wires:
  fq/1 -> Gain/1  "fq"
  Gain/1 -> Data Type Duplicate/2, Divide/2
  Divide/1 -> nStep/1  "nStep"
  Constant/1 -> Data Type Conversion/1
  Data Type Conversion/1 -> Data Type Duplicate/1, Divide/1

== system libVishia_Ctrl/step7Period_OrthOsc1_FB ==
  In1 : Inport  OutDataTypeStr=single
  Constant : Constant  Value=2*pi  OutDataTypeStr=single
  Divide : Product  Inputs=*/
  Real-Imag to Complex : RealImagToComplex
  Trigonometric Function : Trigonometry  Operator=cos
  Trigonometric Function1 : Trigonometry
  Out1 : Outport
  Out2 : Outport  Port=2
  Out3 : Outport  Port=3
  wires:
  Constant/1 -> Divide/1
  Divide/1 -> Trigonometric Function/1, Trigonometric Function1/1, Out3/1  "d"
  In1/1 -> Divide/2  "step7period"
  Real-Imag to Complex/1 -> Out1/1  "fSOO"
  Trigonometric Function1/1 -> Out2/1, Real-Imag to Complex/2  "fSOO1"
  Trigonometric Function/1 -> Real-Imag to Complex/1
